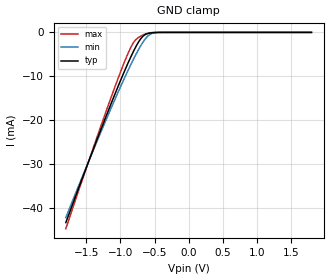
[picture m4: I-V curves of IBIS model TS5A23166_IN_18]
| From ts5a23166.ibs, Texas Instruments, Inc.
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[Model]   TS5A23166_IN_18
Model_type  Input
Vinl=0.6
Vinh=1.5
| variable   typ   min   max
C_comp   1.68pF   1.42pF   1.95pF
[Temperature Range]   40   100   -40
| Ambient temperature   25   85   -40
[Voltage range]   1.8   1.65   1.95
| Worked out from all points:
|   GND clamp passes 1 mA (typ) near -0.68 V on its own axis
[GND Clamp]
| TS5A23166_IN_18
|   Voltage   I(typ)   I(min)   I(max)
-1.8V     -43.4mA    -42.26mA   -44.78mA
-1.355V   -24.96mA   -25.29mA   -24.45mA
-1.04V    -12.55mA   -13.86mA   -10.75mA
-935mV    -8.664mA   -10.24mA   -6.529mA
-860mV    -6.031mA   -7.757mA   -3.819mA
-805mV    -4.228mA   -6.014mA   -2.259mA
-755mV    -2.746mA   -4.512mA   -1.398mA
-680mV    -1.053mA   -2.488mA   -670.8uA
-610mV    -320.4uA   -1.034mA   -241.2uA
-555mV    -115.3uA   -361.1uA   -73.86uA
-485mV    -24.64uA   -62.54uA   -10.21uA
1.8V      32.66pA    93.06pA    21.64pA
